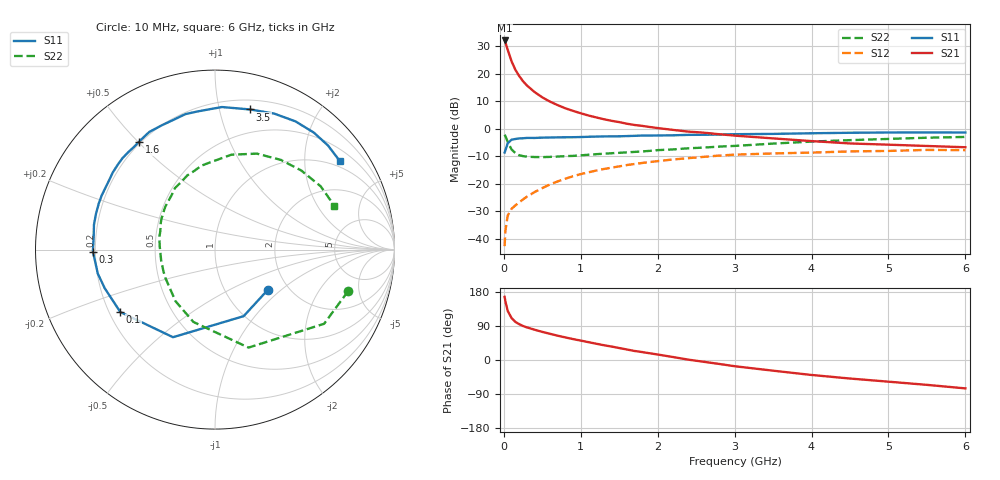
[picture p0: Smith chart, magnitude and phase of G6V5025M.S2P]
! SIEMENS Small Signal Semiconductors
! BFG193
! Si NPN RF Bipolar Junction Transistor in SOT223
! VCE = 0.5 V  IC = 25 mA
! Common Emitter S-Parameters:  August  1996
# GHz  S  MA  R  50
!  f  S11  S21  S12  S22
! GHz  MAG  ANG  MAG  ANG  MAG  ANG  MAG  ANG
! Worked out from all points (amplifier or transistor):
!   36 points, 10 MHz to 6 GHz, reference 50 ohm
!   highest |S21| = 32.0 dB at 10 MHz (marker M1)
!   |S21| within 3 dB of that: start of sweep to 45.8 MHz
!   unconditionally stable (mu >= 1): 355.2 MHz to end of sweep
!   at 250 MHz: K = 0.90, MSG = 21.4 dB, |S12| = -25.6 dB
!   at 1.4 GHz: K = 1.14, MAG = 6.3 dB, |S12| = -14.1 dB
!   at 6 GHz: K = 1.04, MAG = -0.7 dB, |S12| = -7.8 dB
!   S11 on the Smith chart (normalised r, x): 10 MHz: 1.58, -0.82; 100 MHz: 0.24, -0.28; 300 MHz: 0.19, -0.01; 1.6 GHz: 0.19, +0.50; 3.5 GHz: 0.28, +1.24; 6 GHz: 0.82, +2.95
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0.01  0.37 -37.2  39.86 166.6  0.0074 80.3  0.7772 -17.3
0.02  0.4037 -66.7  36.98 155.1  0.014 70.0  0.7351 -34.2
0.05  0.5413 -115.6  27 129.8  0.0265 53.2  0.577 -71.1
0.1  0.6319 -146.6  16.76 110.8  0.0353 46.2  0.4208 -106.6
0.15  0.651 -160.7  11.71 100.5  0.0406 45.6  0.3618 -127.5
0.2  0.6665 -168.4  9.013 94.5  0.0462 48.0  0.3299 -140.0
0.25  0.6711 -174.3  7.238 89.7  0.0523 50.2  0.318 -150.7
0.3  0.6805 -179.0  6.089 86.0  0.0585 51.9  0.3113 -157.5
0.4  0.6796 174.0  4.619 79.9  0.0709 54.1  0.306 -168.6
0.5  0.6883 168.5  3.701 74.2  0.0838 54.4  0.3047 -176.7
0.6  0.6923 163.4  3.1 69.1  0.0975 54.2  0.3083 177.0
0.7  0.6966 158.5  2.675 64.1  0.1106 53.4  0.3124 171.6
0.8  0.6997 154.6  2.343 59.6  0.1239 51.8  0.3182 166.4
1.1  0.7135 143.0  1.735 47.1  0.1617 46.5  0.3369 153.7
1.3  0.7245 135.4  1.485 39.0  0.1858 42.3  0.3512 145.5
1.6  0.7349 125.2  1.23 27.7  0.2191 35.0  0.3726 135.6
2.2  0.7591 107.7  0.951 7.8  0.2764 20.1  0.4207 116.8
2.8  0.7832 91.9  0.794 -10.4  0.3254 5.5  0.4736 99.2
3.5  0.805 75.9  0.667 -28.2  0.356 -12.3  0.5369 80.1
4.5  0.8435 57.9  0.54 -48.9  0.3875 -31.1  0.62 53.7
5.5  0.856 42.6  0.486 -65.6  0.4124 -52.4  0.6864 30.9
6  0.8528 35.2  0.461 -74.9  0.4083 -64.5  0.7087 20.1
